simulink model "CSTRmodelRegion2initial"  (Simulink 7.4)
settings: Solver=ode15s  StartTime=0.0  StopTime=500  RelTol=1e-6
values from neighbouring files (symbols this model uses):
  cain = 2    [runDynSim321.m]    (also in sf_CSTR.m = cInVec(1))
  cbin = 1.5    [runDynSim321.m]    (also in sf_CSTR.m = cInVec(2))
undefined symbols (not defined in the file or in its folder): Floor, Ideal, internal, PI, sigbuilder_block
libraries: simulink_extras x2

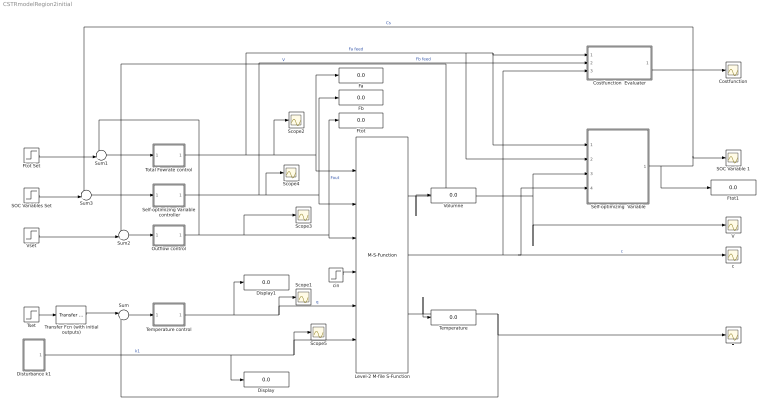
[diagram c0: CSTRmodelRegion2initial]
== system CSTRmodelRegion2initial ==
  Costfunction : Scope
  Costfunction  Evaluater : Subsystem
  Display : Display
  Display1 : Display
  Disturbance k1 : Subsystem
  Fa : Display
  Fb : Display
  Ftot : Display
  Ftot Set : Step  Time=0  Before=22  After=22  SampleTime=0
  Ftot1 : Display
  Level-2 M-file S-Function : M-S-Function  FunctionName=sf_CSTR
  Outflow control : Subsystem  AncestorBlock=simulink/Continuous/PID Controller  DialogController=pidpack.PIDConfig.pidDDGCreate  DialogControllerArgs=DataTag2  mask(PID 1dof){Controller=PI, TimeDomain=Continuous-time, SampleTime=1, IntegratorMethod=Forward Euler, FilterMethod=Forward Euler, Form=Ideal, P=-5, I=0.8, D=0, N=100, InitialConditionSource=internal, InitialConditionForIntegrator=0, InitialConditionForFilter=0, ExternalReset=none, IgnoreLimit=off, ZeroCross=on, LimitOutput=off, UpperSaturationLimit=inf, LowerSaturationLimit=-inf, LinearizeAsGain=off, AntiWindupMode=none, Kb=1, TrackingMode=off, Kt=1, RndMeth=Floor, SaturateOnIntegerOverflow=off, LockScale=off, PParamMin=[], PParamMax=[], PParamDataTypeStr=Inherit: Inherit via internal rule, IParamMin=[], IParamMax=[], IParamDataTypeStr=Inherit: Inherit via internal rule, DParamMin=[], DParamMax=[], DParamDataTypeStr=Inherit: Inherit via internal rule, NParamMin=[], NParamMax=[], NParamDataTypeStr=Inherit: Inherit via internal rule, KbParamMin=[], KbParamMax=[], KbParamDataTypeStr=Inherit: Inherit via internal rule, KtParamMin=[], KtParamMax=[], KtParamDataTypeStr=Inherit: Inherit via internal rule, POutMin=[], POutMax=[], POutDataTypeStr=Inherit: Inherit via internal rule, IOutMin=[], IOutMax=[], IOutDataTypeStr=Inherit: Inherit via internal rule, DOutMin=[], DOutMax=[], DOutDataTypeStr=Inherit: Inherit via internal rule, NOutMin=[], NOutMax=[], NOutDataTypeStr=Inherit: Inherit via internal rule, KbOutMin=[], KbOutMax=[], KbOutDataTypeStr=Inherit: Inherit via internal rule, KtOutMin=[], KtOutMax=[], KtOutDataTypeStr=Inherit: Inherit via internal rule, IntegratorOutMin=[], IntegratorOutMax=[], IntegratorOutDataTypeStr=Inherit: Inherit via internal rule, FilterOutMin=[], FilterOutMax=[], FilterOutDataTypeStr=Inherit: Inherit via internal rule, SumOutMin=[], SumOutMax=[], SumOutDataTypeStr=Inherit: Inherit via internal rule, SumI1OutMin=[], SumI1OutMax=[], SumI1OutDataTypeStr=Inherit: Inherit via internal rule, SumI2OutMin=[], SumI2OutMax=[], SumI2OutDataTypeStr=Inherit: Inherit via internal rule, SumI3OutMin=[], SumI3OutMax=[], SumI3OutDataTypeStr=Inherit: Inherit via internal rule, SumDOutMin=[], SumDOutMax=[], SumDOutDataTypeStr=Inherit: Inherit via internal rule, SumAccumDataTypeStr=Inherit: Inherit via internal rule, SumI1AccumDataTypeStr=Inherit: Inherit via internal rule, SumI2AccumDataTypeStr=Inherit: Inherit via internal rule, SumI3AccumDataTypeStr=Inherit: Inherit via internal rule, SumDAccumDataTypeStr=Inherit: Inherit via internal rule, SaturationOutMin=[], SaturationOutMax=[], SaturationOutDataTypeStr=Inherit: Same as input, IntegratorContinuousStateAttributes='', IntegratorStateIdentifier=, IntegratorStateMustResolveToSignalObject=off, IntegratorRTWStateStorageClass=Auto, IntegratorRTWStateStorageTypeQualifier=, FilterContinuousStateAttributes='', FilterStateIdentifier=, FilterStateMustResolveToSignalObject=off, FilterRTWStateStorageClass=Auto, FilterRTWStateStorageTypeQualifier=}
      mask prompts: TimeDomain "Time-domain:"; SampleTime "Sample time (-1 for inherited):"; IntegratorMethod "Integrator method:"; FilterMethod "Filter method:"; Form "Controller form:"; P "Proportional (P):"; I "Integral (I):"; D "Derivative (D):"; N "Filter coefficient (N):"; InitialConditionSource "Source:"; InitialConditionForIntegrator "Integrator:"; InitialConditionForFilter "Filter:"; ExternalReset "External reset:"; IgnoreLimit "Ignore reset when linearizing"; ZeroCross "Enable zero-crossing detection"; LimitOutput "Limit output"; UpperSaturationLimit "Upper saturation limit:"; LowerSaturationLimit "Lower saturation limit:"; LinearizeAsGain "Ignore saturation when linearizing"; AntiWindupMode "Anti-windup method:"; Kb "Back-calculation coefficient (Kb):"; TrackingMode "Enable tracking mode"; Kt "Tracking coefficient (Kt):"; RndMeth "Integer rounding mode:"; SaturateOnIntegerOverflow "Saturate on integer overflow"; LockScale "Lock data type settings against changes by the fixed-point tools"; PParamMin "P parameter minimum:"; PParamMax "P parameter maximum:"; PParamDataTypeStr "P parameter:"; IParamMin "I parameter minimum:"; IParamMax "I parameter maximum:"; IParamDataTypeStr "I parameter:"; DParamMin "D parameter minimum:"; DParamMax "D parameter maximum:"; DParamDataTypeStr "D parameter:"; NParamMin "N parameter minimum:"; NParamMax "N parameter maximum:"; NParamDataTypeStr "N parameter:"; KbParamMin "Kb parameter minimum:"; KbParamMax "Kb parameter maximum:"; KbParamDataTypeStr "Kb parameter:"; KtParamMin "Kt parameter minimum:"; KtParamMax "Kt parameter maximum:"; KtParamDataTypeStr "Kt parameter:"; POutMin "P product output minimum:"; POutMax "P product output maximum:"; POutDataTypeStr "P product output:"; IOutMin "I product output minimum:"; IOutMax "I product output maximum:"; IOutDataTypeStr "I product output:"; DOutMin "D product output minimum:"; DOutMax "D product output maximum:"; DOutDataTypeStr "D product output:"; NOutMin "N product output minimum:"; NOutMax "N product output maximum:"; NOutDataTypeStr "N product output:"; KbOutMin "Kb product output minimum:"; KbOutMax "Kb product output maximum:"; KbOutDataTypeStr "Kb product output:"; KtOutMin "Kt product output minimum:"; KtOutMax "Kt product output maximum:"; KtOutDataTypeStr "Kt product output:"; IntegratorOutMin "Integrator output minimum:"; IntegratorOutMax "Integrator output maximum:"; IntegratorOutDataTypeStr "Integrator output:"; FilterOutMin "Filter output minimum:"; FilterOutMax "Filter output maximum:"; FilterOutDataTypeStr "Filter output:"; SumOutMin "Sum output minimum:"; SumOutMax "Sum output maximum:"; SumOutDataTypeStr "Sum output:"; SumI1OutMin "SumI1 output minimum:"; SumI1OutMax "SumI1 output maximum:"; SumI1OutDataTypeStr "SumI1 output:"; SumI2OutMin "SumI2 output minimum:"; SumI2OutMax "SumI2 output maximum:"; SumI2OutDataTypeStr "SumI2 output:"; SumI3OutMin "SumI3 output minimum:"; SumI3OutMax "SumI3 output maximum:"; SumI3OutDataTypeStr "SumI3 output:"; SumDOutMin "SumD output minimum:"; SumDOutMax "SumD output maximum:"; SumDOutDataTypeStr "SumD output:"; SumAccumDataTypeStr "Accumulator of Sum:"; SumI1AccumDataTypeStr "Accumulator of SumI1:"; SumI2AccumDataTypeStr "Accumulator of SumI2:"; SumI3AccumDataTypeStr "Accumulator of SumI3:"; SumDAccumDataTypeStr "Accumulator of SumD:"; SaturationOutMin "Saturation output minimum:"; SaturationOutMax "Saturation output maximum:"; SaturationOutDataTypeStr "Saturation output:"; IntegratorContinuousStateAttributes "State name: (e.g., 'position')"; IntegratorStateIdentifier "State name:"; IntegratorStateMustResolveToSignalObject "State name must resolve to Simulink signal object"; IntegratorRTWStateStorageClass "Real-Time Workshop storage class:"; IntegratorRTWStateStorageTypeQualifier "Real-Time Workshop storage type qualifier:"; FilterContinuousStateAttributes "State name: (e.g., 'position')"; FilterStateIdentifier "State name:"; FilterStateMustResolveToSignalObject "State name must resolve to Simulink signal object"; FilterRTWStateStorageClass "Real-Time Workshop storage class:"; FilterRTWStateStorageTypeQualifier "Real-Time Workshop storage type qualifier:"
      mask help: This block implements continuous- and discrete-time PID control algorithms and includes advanced features such as anti-windup, external reset, and signal tracking. You can tune the PID gains automatically using the 'Tune...' button (requires Simulink Control Design).
      mask init:
      | [shiftx shifty satshiftx satshifty] = pidpack.PIDConfig.configPID(gcbh);
  SOC Variable 1 : Scope
  SOC Variables Set : Step  Time=0  After=0  SampleTime=0
  Scope{1..5} (5 alike) : Scope
  Self-optimizing  Variable : Stateflow chart
  Self-optimizing Variable  controller : Subsystem  AncestorBlock=simulink/Continuous/PID Controller  DialogController=pidpack.PIDConfig.pidDDGCreate  DialogControllerArgs=DataTag3  mask(PID 1dof){Controller=PI, TimeDomain=Continuous-time, SampleTime=1, IntegratorMethod=Forward Euler, FilterMethod=Forward Euler, Form=Ideal, P=145, I=3, D=0, N=100, InitialConditionSource=internal, InitialConditionForIntegrator=0, InitialConditionForFilter=0, ExternalReset=none, IgnoreLimit=off, ZeroCross=on, LimitOutput=off, UpperSaturationLimit=1e6, LowerSaturationLimit=0, LinearizeAsGain=off, AntiWindupMode=none, Kb=1, TrackingMode=off, Kt=1, RndMeth=Floor, SaturateOnIntegerOverflow=off, LockScale=off, PParamMin=[], PParamMax=[], PParamDataTypeStr=Inherit: Inherit via internal rule, IParamMin=[], IParamMax=[], IParamDataTypeStr=Inherit: Inherit via internal rule, DParamMin=[], DParamMax=[], DParamDataTypeStr=Inherit: Inherit via internal rule, NParamMin=[], NParamMax=[], NParamDataTypeStr=Inherit: Inherit via internal rule, KbParamMin=[], KbParamMax=[], KbParamDataTypeStr=Inherit: Inherit via internal rule, KtParamMin=[], KtParamMax=[], KtParamDataTypeStr=Inherit: Inherit via internal rule, POutMin=[], POutMax=[], POutDataTypeStr=Inherit: Inherit via internal rule, IOutMin=[], IOutMax=[], IOutDataTypeStr=Inherit: Inherit via internal rule, DOutMin=[], DOutMax=[], DOutDataTypeStr=Inherit: Inherit via internal rule, NOutMin=[], NOutMax=[], NOutDataTypeStr=Inherit: Inherit via internal rule, KbOutMin=[], KbOutMax=[], KbOutDataTypeStr=Inherit: Inherit via internal rule, KtOutMin=[], KtOutMax=[], KtOutDataTypeStr=Inherit: Inherit via internal rule, IntegratorOutMin=[], IntegratorOutMax=[], IntegratorOutDataTypeStr=Inherit: Inherit via internal rule, FilterOutMin=[], FilterOutMax=[], FilterOutDataTypeStr=Inherit: Inherit via internal rule, SumOutMin=[], SumOutMax=[], SumOutDataTypeStr=Inherit: Inherit via internal rule, SumI1OutMin=[], SumI1OutMax=[], SumI1OutDataTypeStr=Inherit: Inherit via internal rule, SumI2OutMin=[], SumI2OutMax=[], SumI2OutDataTypeStr=Inherit: Inherit via internal rule, SumI3OutMin=[], SumI3OutMax=[], SumI3OutDataTypeStr=Inherit: Inherit via internal rule, SumDOutMin=[], SumDOutMax=[], SumDOutDataTypeStr=Inherit: Inherit via internal rule, SumAccumDataTypeStr=Inherit: Inherit via internal rule, SumI1AccumDataTypeStr=Inherit: Inherit via internal rule, SumI2AccumDataTypeStr=Inherit: Inherit via internal rule, SumI3AccumDataTypeStr=Inherit: Inherit via internal rule, SumDAccumDataTypeStr=Inherit: Inherit via internal rule, SaturationOutMin=[], SaturationOutMax=[], SaturationOutDataTypeStr=Inherit: Same as input, IntegratorContinuousStateAttributes='', IntegratorStateIdentifier=, IntegratorStateMustResolveToSignalObject=off, IntegratorRTWStateStorageClass=Auto, IntegratorRTWStateStorageTypeQualifier=, FilterContinuousStateAttributes='', FilterStateIdentifier=, FilterStateMustResolveToSignalObject=off, FilterRTWStateStorageClass=Auto, FilterRTWStateStorageTypeQualifier=}
      mask prompts: TimeDomain "Time-domain:"; SampleTime "Sample time (-1 for inherited):"; IntegratorMethod "Integrator method:"; FilterMethod "Filter method:"; Form "Controller form:"; P "Proportional (P):"; I "Integral (I):"; D "Derivative (D):"; N "Filter coefficient (N):"; InitialConditionSource "Source:"; InitialConditionForIntegrator "Integrator:"; InitialConditionForFilter "Filter:"; ExternalReset "External reset:"; IgnoreLimit "Ignore reset when linearizing"; ZeroCross "Enable zero-crossing detection"; LimitOutput "Limit output"; UpperSaturationLimit "Upper saturation limit:"; LowerSaturationLimit "Lower saturation limit:"; LinearizeAsGain "Ignore saturation when linearizing"; AntiWindupMode "Anti-windup method:"; Kb "Back-calculation coefficient (Kb):"; TrackingMode "Enable tracking mode"; Kt "Tracking coefficient (Kt):"; RndMeth "Integer rounding mode:"; SaturateOnIntegerOverflow "Saturate on integer overflow"; LockScale "Lock data type settings against changes by the fixed-point tools"; PParamMin "P parameter minimum:"; PParamMax "P parameter maximum:"; PParamDataTypeStr "P parameter:"; IParamMin "I parameter minimum:"; IParamMax "I parameter maximum:"; IParamDataTypeStr "I parameter:"; DParamMin "D parameter minimum:"; DParamMax "D parameter maximum:"; DParamDataTypeStr "D parameter:"; NParamMin "N parameter minimum:"; NParamMax "N parameter maximum:"; NParamDataTypeStr "N parameter:"; KbParamMin "Kb parameter minimum:"; KbParamMax "Kb parameter maximum:"; KbParamDataTypeStr "Kb parameter:"; KtParamMin "Kt parameter minimum:"; KtParamMax "Kt parameter maximum:"; KtParamDataTypeStr "Kt parameter:"; POutMin "P product output minimum:"; POutMax "P product output maximum:"; POutDataTypeStr "P product output:"; IOutMin "I product output minimum:"; IOutMax "I product output maximum:"; IOutDataTypeStr "I product output:"; DOutMin "D product output minimum:"; DOutMax "D product output maximum:"; DOutDataTypeStr "D product output:"; NOutMin "N product output minimum:"; NOutMax "N product output maximum:"; NOutDataTypeStr "N product output:"; KbOutMin "Kb product output minimum:"; KbOutMax "Kb product output maximum:"; KbOutDataTypeStr "Kb product output:"; KtOutMin "Kt product output minimum:"; KtOutMax "Kt product output maximum:"; KtOutDataTypeStr "Kt product output:"; IntegratorOutMin "Integrator output minimum:"; IntegratorOutMax "Integrator output maximum:"; IntegratorOutDataTypeStr "Integrator output:"; FilterOutMin "Filter output minimum:"; FilterOutMax "Filter output maximum:"; FilterOutDataTypeStr "Filter output:"; SumOutMin "Sum output minimum:"; SumOutMax "Sum output maximum:"; SumOutDataTypeStr "Sum output:"; SumI1OutMin "SumI1 output minimum:"; SumI1OutMax "SumI1 output maximum:"; SumI1OutDataTypeStr "SumI1 output:"; SumI2OutMin "SumI2 output minimum:"; SumI2OutMax "SumI2 output maximum:"; SumI2OutDataTypeStr "SumI2 output:"; SumI3OutMin "SumI3 output minimum:"; SumI3OutMax "SumI3 output maximum:"; SumI3OutDataTypeStr "SumI3 output:"; SumDOutMin "SumD output minimum:"; SumDOutMax "SumD output maximum:"; SumDOutDataTypeStr "SumD output:"; SumAccumDataTypeStr "Accumulator of Sum:"; SumI1AccumDataTypeStr "Accumulator of SumI1:"; SumI2AccumDataTypeStr "Accumulator of SumI2:"; SumI3AccumDataTypeStr "Accumulator of SumI3:"; SumDAccumDataTypeStr "Accumulator of SumD:"; SaturationOutMin "Saturation output minimum:"; SaturationOutMax "Saturation output maximum:"; SaturationOutDataTypeStr "Saturation output:"; IntegratorContinuousStateAttributes "State name: (e.g., 'position')"; IntegratorStateIdentifier "State name:"; IntegratorStateMustResolveToSignalObject "State name must resolve to Simulink signal object"; IntegratorRTWStateStorageClass "Real-Time Workshop storage class:"; IntegratorRTWStateStorageTypeQualifier "Real-Time Workshop storage type qualifier:"; FilterContinuousStateAttributes "State name: (e.g., 'position')"; FilterStateIdentifier "State name:"; FilterStateMustResolveToSignalObject "State name must resolve to Simulink signal object"; FilterRTWStateStorageClass "Real-Time Workshop storage class:"; FilterRTWStateStorageTypeQualifier "Real-Time Workshop storage type qualifier:"
      mask help: This block implements continuous- and discrete-time PID control algorithms and includes advanced features such as anti-windup, external reset, and signal tracking. You can tune the PID gains automatically using the 'Tune...' button (requires Simulink Control Design).
      mask init:
      | [shiftx shifty satshiftx satshifty] = pidpack.PIDConfig.configPID(gcbh);
  Sum : Sum  Inputs=|+-  OutDataType=fixdt(1, 16)  OutScaling=2^0
  Sum1 : Sum  Inputs=-+|  OutDataType=fixdt(1, 16)  OutScaling=2^0
  Sum2 : Sum  Inputs=-+|  OutDataType=fixdt(1, 16)  OutScaling=2^0
  Sum3 : Sum  Inputs=-+|  OutDataType=fixdt(1, 16)  OutScaling=2^0
  T : Scope
  Temperature : Display
  Temperature control : Subsystem  AncestorBlock=simulink/Continuous/PID Controller  DialogController=pidpack.PIDConfig.pidDDGCreate  DialogControllerArgs=DataTag4  mask(PID 1dof){Controller=PI, TimeDomain=Continuous-time, SampleTime=1, IntegratorMethod=Forward Euler, FilterMethod=Forward Euler, Form=Ideal, P=-3521, I=2.4, D=0, N=100, InitialConditionSource=internal, InitialConditionForIntegrator=888, InitialConditionForFilter=0, ExternalReset=none, IgnoreLimit=off, ZeroCross=on, LimitOutput=off, UpperSaturationLimit=1e3, LowerSaturationLimit=0, LinearizeAsGain=off, AntiWindupMode=none, Kb=1, TrackingMode=off, Kt=1, RndMeth=Floor, SaturateOnIntegerOverflow=off, LockScale=off, PParamMin=[], PParamMax=[], PParamDataTypeStr=Inherit: Inherit via internal rule, IParamMin=[], IParamMax=[], IParamDataTypeStr=Inherit: Inherit via internal rule, DParamMin=[], DParamMax=[], DParamDataTypeStr=Inherit: Inherit via internal rule, NParamMin=[], NParamMax=[], NParamDataTypeStr=Inherit: Inherit via internal rule, KbParamMin=[], KbParamMax=[], KbParamDataTypeStr=Inherit: Inherit via internal rule, KtParamMin=[], KtParamMax=[], KtParamDataTypeStr=Inherit: Inherit via internal rule, POutMin=[], POutMax=[], POutDataTypeStr=Inherit: Inherit via internal rule, IOutMin=[], IOutMax=[], IOutDataTypeStr=Inherit: Inherit via internal rule, DOutMin=[], DOutMax=[], DOutDataTypeStr=Inherit: Inherit via internal rule, NOutMin=[], NOutMax=[], NOutDataTypeStr=Inherit: Inherit via internal rule, KbOutMin=[], KbOutMax=[], KbOutDataTypeStr=Inherit: Inherit via internal rule, KtOutMin=[], KtOutMax=[], KtOutDataTypeStr=Inherit: Inherit via internal rule, IntegratorOutMin=[], IntegratorOutMax=[], IntegratorOutDataTypeStr=Inherit: Inherit via internal rule, FilterOutMin=[], FilterOutMax=[], FilterOutDataTypeStr=Inherit: Inherit via internal rule, SumOutMin=[], SumOutMax=[], SumOutDataTypeStr=Inherit: Inherit via internal rule, SumI1OutMin=[], SumI1OutMax=[], SumI1OutDataTypeStr=Inherit: Inherit via internal rule, SumI2OutMin=[], SumI2OutMax=[], SumI2OutDataTypeStr=Inherit: Inherit via internal rule, SumI3OutMin=[], SumI3OutMax=[], SumI3OutDataTypeStr=Inherit: Inherit via internal rule, SumDOutMin=[], SumDOutMax=[], SumDOutDataTypeStr=Inherit: Inherit via internal rule, SumAccumDataTypeStr=Inherit: Inherit via internal rule, SumI1AccumDataTypeStr=Inherit: Inherit via internal rule, SumI2AccumDataTypeStr=Inherit: Inherit via internal rule, SumI3AccumDataTypeStr=Inherit: Inherit via internal rule, SumDAccumDataTypeStr=Inherit: Inherit via internal rule, SaturationOutMin=[], SaturationOutMax=[], SaturationOutDataTypeStr=Inherit: Same as input, IntegratorContinuousStateAttributes='', IntegratorStateIdentifier=, IntegratorStateMustResolveToSignalObject=off, IntegratorRTWStateStorageClass=Auto, IntegratorRTWStateStorageTypeQualifier=, FilterContinuousStateAttributes='', FilterStateIdentifier=, FilterStateMustResolveToSignalObject=off, FilterRTWStateStorageClass=Auto, FilterRTWStateStorageTypeQualifier=}
      mask prompts: TimeDomain "Time-domain:"; SampleTime "Sample time (-1 for inherited):"; IntegratorMethod "Integrator method:"; FilterMethod "Filter method:"; Form "Controller form:"; P "Proportional (P):"; I "Integral (I):"; D "Derivative (D):"; N "Filter coefficient (N):"; InitialConditionSource "Source:"; InitialConditionForIntegrator "Integrator:"; InitialConditionForFilter "Filter:"; ExternalReset "External reset:"; IgnoreLimit "Ignore reset when linearizing"; ZeroCross "Enable zero-crossing detection"; LimitOutput "Limit output"; UpperSaturationLimit "Upper saturation limit:"; LowerSaturationLimit "Lower saturation limit:"; LinearizeAsGain "Ignore saturation when linearizing"; AntiWindupMode "Anti-windup method:"; Kb "Back-calculation coefficient (Kb):"; TrackingMode "Enable tracking mode"; Kt "Tracking coefficient (Kt):"; RndMeth "Integer rounding mode:"; SaturateOnIntegerOverflow "Saturate on integer overflow"; LockScale "Lock data type settings against changes by the fixed-point tools"; PParamMin "P parameter minimum:"; PParamMax "P parameter maximum:"; PParamDataTypeStr "P parameter:"; IParamMin "I parameter minimum:"; IParamMax "I parameter maximum:"; IParamDataTypeStr "I parameter:"; DParamMin "D parameter minimum:"; DParamMax "D parameter maximum:"; DParamDataTypeStr "D parameter:"; NParamMin "N parameter minimum:"; NParamMax "N parameter maximum:"; NParamDataTypeStr "N parameter:"; KbParamMin "Kb parameter minimum:"; KbParamMax "Kb parameter maximum:"; KbParamDataTypeStr "Kb parameter:"; KtParamMin "Kt parameter minimum:"; KtParamMax "Kt parameter maximum:"; KtParamDataTypeStr "Kt parameter:"; POutMin "P product output minimum:"; POutMax "P product output maximum:"; POutDataTypeStr "P product output:"; IOutMin "I product output minimum:"; IOutMax "I product output maximum:"; IOutDataTypeStr "I product output:"; DOutMin "D product output minimum:"; DOutMax "D product output maximum:"; DOutDataTypeStr "D product output:"; NOutMin "N product output minimum:"; NOutMax "N product output maximum:"; NOutDataTypeStr "N product output:"; KbOutMin "Kb product output minimum:"; KbOutMax "Kb product output maximum:"; KbOutDataTypeStr "Kb product output:"; KtOutMin "Kt product output minimum:"; KtOutMax "Kt product output maximum:"; KtOutDataTypeStr "Kt product output:"; IntegratorOutMin "Integrator output minimum:"; IntegratorOutMax "Integrator output maximum:"; IntegratorOutDataTypeStr "Integrator output:"; FilterOutMin "Filter output minimum:"; FilterOutMax "Filter output maximum:"; FilterOutDataTypeStr "Filter output:"; SumOutMin "Sum output minimum:"; SumOutMax "Sum output maximum:"; SumOutDataTypeStr "Sum output:"; SumI1OutMin "SumI1 output minimum:"; SumI1OutMax "SumI1 output maximum:"; SumI1OutDataTypeStr "SumI1 output:"; SumI2OutMin "SumI2 output minimum:"; SumI2OutMax "SumI2 output maximum:"; SumI2OutDataTypeStr "SumI2 output:"; SumI3OutMin "SumI3 output minimum:"; SumI3OutMax "SumI3 output maximum:"; SumI3OutDataTypeStr "SumI3 output:"; SumDOutMin "SumD output minimum:"; SumDOutMax "SumD output maximum:"; SumDOutDataTypeStr "SumD output:"; SumAccumDataTypeStr "Accumulator of Sum:"; SumI1AccumDataTypeStr "Accumulator of SumI1:"; SumI2AccumDataTypeStr "Accumulator of SumI2:"; SumI3AccumDataTypeStr "Accumulator of SumI3:"; SumDAccumDataTypeStr "Accumulator of SumD:"; SaturationOutMin "Saturation output minimum:"; SaturationOutMax "Saturation output maximum:"; SaturationOutDataTypeStr "Saturation output:"; IntegratorContinuousStateAttributes "State name: (e.g., 'position')"; IntegratorStateIdentifier "State name:"; IntegratorStateMustResolveToSignalObject "State name must resolve to Simulink signal object"; IntegratorRTWStateStorageClass "Real-Time Workshop storage class:"; IntegratorRTWStateStorageTypeQualifier "Real-Time Workshop storage type qualifier:"; FilterContinuousStateAttributes "State name: (e.g., 'position')"; FilterStateIdentifier "State name:"; FilterStateMustResolveToSignalObject "State name must resolve to Simulink signal object"; FilterRTWStateStorageClass "Real-Time Workshop storage class:"; FilterRTWStateStorageTypeQualifier "Real-Time Workshop storage type qualifier:"
      mask help: This block implements continuous- and discrete-time PID control algorithms and includes advanced features such as anti-windup, external reset, and signal tracking. You can tune the PID gains automatically using the 'Tune...' button (requires Simulink Control Design).
      mask init:
      | [shiftx shifty satshiftx satshifty] = pidpack.PIDConfig.configPID(gcbh);
  Total Fowrate control : Subsystem  AncestorBlock=simulink/Continuous/PID Controller  DialogController=pidpack.PIDConfig.pidDDGCreate  DialogControllerArgs=DataTag5  mask(PID 1dof){Controller=PI, TimeDomain=Continuous-time, SampleTime=1, IntegratorMethod=Forward Euler, FilterMethod=Forward Euler, Form=Ideal, P=0.58, I=0.35, D=0, N=100, InitialConditionSource=internal, InitialConditionForIntegrator=0, InitialConditionForFilter=0, ExternalReset=none, IgnoreLimit=off, ZeroCross=on, LimitOutput=off, UpperSaturationLimit=1e6, LowerSaturationLimit=0, LinearizeAsGain=off, AntiWindupMode=none, Kb=1, TrackingMode=off, Kt=1, RndMeth=Floor, SaturateOnIntegerOverflow=off, LockScale=off, PParamMin=[], PParamMax=[], PParamDataTypeStr=Inherit: Inherit via internal rule, IParamMin=[], IParamMax=[], IParamDataTypeStr=Inherit: Inherit via internal rule, DParamMin=[], DParamMax=[], DParamDataTypeStr=Inherit: Inherit via internal rule, NParamMin=[], NParamMax=[], NParamDataTypeStr=Inherit: Inherit via internal rule, KbParamMin=[], KbParamMax=[], KbParamDataTypeStr=Inherit: Inherit via internal rule, KtParamMin=[], KtParamMax=[], KtParamDataTypeStr=Inherit: Inherit via internal rule, POutMin=[], POutMax=[], POutDataTypeStr=Inherit: Inherit via internal rule, IOutMin=[], IOutMax=[], IOutDataTypeStr=Inherit: Inherit via internal rule, DOutMin=[], DOutMax=[], DOutDataTypeStr=Inherit: Inherit via internal rule, NOutMin=[], NOutMax=[], NOutDataTypeStr=Inherit: Inherit via internal rule, KbOutMin=[], KbOutMax=[], KbOutDataTypeStr=Inherit: Inherit via internal rule, KtOutMin=[], KtOutMax=[], KtOutDataTypeStr=Inherit: Inherit via internal rule, IntegratorOutMin=[], IntegratorOutMax=[], IntegratorOutDataTypeStr=Inherit: Inherit via internal rule, FilterOutMin=[], FilterOutMax=[], FilterOutDataTypeStr=Inherit: Inherit via internal rule, SumOutMin=[], SumOutMax=[], SumOutDataTypeStr=Inherit: Inherit via internal rule, SumI1OutMin=[], SumI1OutMax=[], SumI1OutDataTypeStr=Inherit: Inherit via internal rule, SumI2OutMin=[], SumI2OutMax=[], SumI2OutDataTypeStr=Inherit: Inherit via internal rule, SumI3OutMin=[], SumI3OutMax=[], SumI3OutDataTypeStr=Inherit: Inherit via internal rule, SumDOutMin=[], SumDOutMax=[], SumDOutDataTypeStr=Inherit: Inherit via internal rule, SumAccumDataTypeStr=Inherit: Inherit via internal rule, SumI1AccumDataTypeStr=Inherit: Inherit via internal rule, SumI2AccumDataTypeStr=Inherit: Inherit via internal rule, SumI3AccumDataTypeStr=Inherit: Inherit via internal rule, SumDAccumDataTypeStr=Inherit: Inherit via internal rule, SaturationOutMin=[], SaturationOutMax=[], SaturationOutDataTypeStr=Inherit: Same as input, IntegratorContinuousStateAttributes='', IntegratorStateIdentifier=, IntegratorStateMustResolveToSignalObject=off, IntegratorRTWStateStorageClass=Auto, IntegratorRTWStateStorageTypeQualifier=, FilterContinuousStateAttributes='', FilterStateIdentifier=, FilterStateMustResolveToSignalObject=off, FilterRTWStateStorageClass=Auto, FilterRTWStateStorageTypeQualifier=}
      mask prompts: TimeDomain "Time-domain:"; SampleTime "Sample time (-1 for inherited):"; IntegratorMethod "Integrator method:"; FilterMethod "Filter method:"; Form "Controller form:"; P "Proportional (P):"; I "Integral (I):"; D "Derivative (D):"; N "Filter coefficient (N):"; InitialConditionSource "Source:"; InitialConditionForIntegrator "Integrator:"; InitialConditionForFilter "Filter:"; ExternalReset "External reset:"; IgnoreLimit "Ignore reset when linearizing"; ZeroCross "Enable zero-crossing detection"; LimitOutput "Limit output"; UpperSaturationLimit "Upper saturation limit:"; LowerSaturationLimit "Lower saturation limit:"; LinearizeAsGain "Ignore saturation when linearizing"; AntiWindupMode "Anti-windup method:"; Kb "Back-calculation coefficient (Kb):"; TrackingMode "Enable tracking mode"; Kt "Tracking coefficient (Kt):"; RndMeth "Integer rounding mode:"; SaturateOnIntegerOverflow "Saturate on integer overflow"; LockScale "Lock data type settings against changes by the fixed-point tools"; PParamMin "P parameter minimum:"; PParamMax "P parameter maximum:"; PParamDataTypeStr "P parameter:"; IParamMin "I parameter minimum:"; IParamMax "I parameter maximum:"; IParamDataTypeStr "I parameter:"; DParamMin "D parameter minimum:"; DParamMax "D parameter maximum:"; DParamDataTypeStr "D parameter:"; NParamMin "N parameter minimum:"; NParamMax "N parameter maximum:"; NParamDataTypeStr "N parameter:"; KbParamMin "Kb parameter minimum:"; KbParamMax "Kb parameter maximum:"; KbParamDataTypeStr "Kb parameter:"; KtParamMin "Kt parameter minimum:"; KtParamMax "Kt parameter maximum:"; KtParamDataTypeStr "Kt parameter:"; POutMin "P product output minimum:"; POutMax "P product output maximum:"; POutDataTypeStr "P product output:"; IOutMin "I product output minimum:"; IOutMax "I product output maximum:"; IOutDataTypeStr "I product output:"; DOutMin "D product output minimum:"; DOutMax "D product output maximum:"; DOutDataTypeStr "D product output:"; NOutMin "N product output minimum:"; NOutMax "N product output maximum:"; NOutDataTypeStr "N product output:"; KbOutMin "Kb product output minimum:"; KbOutMax "Kb product output maximum:"; KbOutDataTypeStr "Kb product output:"; KtOutMin "Kt product output minimum:"; KtOutMax "Kt product output maximum:"; KtOutDataTypeStr "Kt product output:"; IntegratorOutMin "Integrator output minimum:"; IntegratorOutMax "Integrator output maximum:"; IntegratorOutDataTypeStr "Integrator output:"; FilterOutMin "Filter output minimum:"; FilterOutMax "Filter output maximum:"; FilterOutDataTypeStr "Filter output:"; SumOutMin "Sum output minimum:"; SumOutMax "Sum output maximum:"; SumOutDataTypeStr "Sum output:"; SumI1OutMin "SumI1 output minimum:"; SumI1OutMax "SumI1 output maximum:"; SumI1OutDataTypeStr "SumI1 output:"; SumI2OutMin "SumI2 output minimum:"; SumI2OutMax "SumI2 output maximum:"; SumI2OutDataTypeStr "SumI2 output:"; SumI3OutMin "SumI3 output minimum:"; SumI3OutMax "SumI3 output maximum:"; SumI3OutDataTypeStr "SumI3 output:"; SumDOutMin "SumD output minimum:"; SumDOutMax "SumD output maximum:"; SumDOutDataTypeStr "SumD output:"; SumAccumDataTypeStr "Accumulator of Sum:"; SumI1AccumDataTypeStr "Accumulator of SumI1:"; SumI2AccumDataTypeStr "Accumulator of SumI2:"; SumI3AccumDataTypeStr "Accumulator of SumI3:"; SumDAccumDataTypeStr "Accumulator of SumD:"; SaturationOutMin "Saturation output minimum:"; SaturationOutMax "Saturation output maximum:"; SaturationOutDataTypeStr "Saturation output:"; IntegratorContinuousStateAttributes "State name: (e.g., 'position')"; IntegratorStateIdentifier "State name:"; IntegratorStateMustResolveToSignalObject "State name must resolve to Simulink signal object"; IntegratorRTWStateStorageClass "Real-Time Workshop storage class:"; IntegratorRTWStateStorageTypeQualifier "Real-Time Workshop storage type qualifier:"; FilterContinuousStateAttributes "State name: (e.g., 'position')"; FilterStateIdentifier "State name:"; FilterStateMustResolveToSignalObject "State name must resolve to Simulink signal object"; FilterRTWStateStorageClass "Real-Time Workshop storage class:"; FilterRTWStateStorageTypeQualifier "Real-Time Workshop storage type qualifier:"
      mask help: This block implements continuous- and discrete-time PID control algorithms and includes advanced features such as anti-windup, external reset, and signal tracking. You can tune the PID gains automatically using the 'Tune...' button (requires Simulink Control Design).
      mask init:
      | [shiftx shifty satshiftx satshifty] = pidpack.PIDConfig.configPID(gcbh);
  Transfer Fcn (with initial outputs) : simulink_extras/Additional Linear/Transfer Fcn (with initial outputs)  SystemSampleTime=-1  N=[1]  D="[10  1]"  Y0=350  U0=0
  Tset : Step  Time=250  Before=350  After=350  SampleTime=0
  V : Scope
  Volumne : Display
  Vset : Step  Time=0  Before=500  After=500  SampleTime=0
  c : Scope
  cin : Step  Time=0  Before=[cain cbin 0 0]  After=[cain cbin 0 0]  SampleTime=0
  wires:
  cin/1 -> Level-2 M-file S-Function/4
  Sum/1 -> Temperature control/1(u)
  Level-2 M-file S-Function/1 -> Sum2/1, Self-optimizing  Variable/3(V), V/1, Volumne/1  "V"
  Level-2 M-file S-Function/2 -> Costfunction  Evaluater/3(Concentrations), c/1, Self-optimizing  Variable/4(cVector)  "c"
  Level-2 M-file S-Function/3 -> T/1, Sum/2, Temperature/1  "T"
  Tset/1 -> Transfer Fcn (with initial outputs)/1
  Vset/1 -> Sum2/2
  Sum2/1 -> Outflow control/1(u)
  Costfunction  Evaluater/1(Objective) -> Costfunction/1
  Outflow control/1(y) -> Scope3/1, Level-2 M-file S-Function/3, Ftot/1, Sum1/1  "Fout"
  Temperature control/1(y) -> Level-2 M-file S-Function/5, Scope1/1, Display1/1  "q"
  Sum1/1 -> Total Fowrate control/1(u)
  Total Fowrate control/1(y) -> Scope2/1, Level-2 M-file S-Function/1, Fa/1, Costfunction  Evaluater/1(Fa), Self-optimizing  Variable/1(Fa), Self-optimizing  Variable/2(Fb)  "Fa feed"
  Self-optimizing  Variable/1(cs) -> SOC Variable 1/1, Sum3/1, Ftot1/1  "Cs"
  SOC Variables Set/1 -> Sum3/2
  Sum3/1 -> Self-optimizing Variable  controller/1(u)
  Self-optimizing Variable  controller/1(y) -> Costfunction  Evaluater/2(Fb), Scope4/1, Level-2 M-file S-Function/2, Fb/1  "Fb feed"
  Ftot Set/1 -> Sum1/2
  Disturbance k1/1(Out1) -> Level-2 M-file S-Function/6, Scope5/1, Display/1  "k1"
  Transfer Fcn (with initial outputs)/1 -> Sum/1

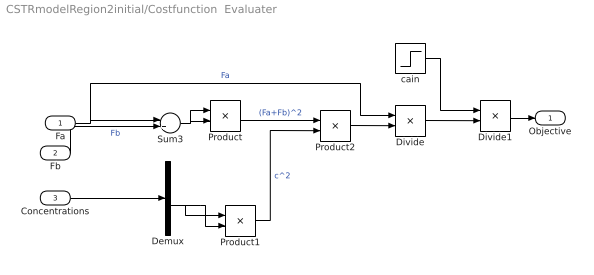
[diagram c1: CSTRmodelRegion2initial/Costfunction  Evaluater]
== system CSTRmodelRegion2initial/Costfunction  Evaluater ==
  Fa : Inport
  Fb : Inport  Port=2
  Concentrations : Inport  Port=3
  Demux : Demux
  Divide : Product  Inputs=/*  OutDataType=fixdt(1, 16)  OutScaling=2^-10
  Divide1 : Product  Inputs=/*  OutDataType=fixdt(1, 16)  OutScaling=2^-10
  Product : Product  OutDataType=fixdt(1, 16)  OutScaling=2^0
  Product1 : Product  OutDataType=fixdt(1, 16)  OutScaling=2^0
  Product2 : Product  OutDataType=fixdt(1, 16)  OutScaling=2^0
  Sum3 : Sum  Inputs=|++  OutDataType=fixdt(1, 16)  OutScaling=2^0
  cain : Step  Before=cain  After=cain  SampleTime=0
  Objective : Outport
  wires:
  Sum3/1 -> Product/1, Product/2
  Demux/3 -> Product1/2, Product1/1
  Product/1 -> Product2/1  "(Fa+Fb)^2"
  Product1/1 -> Product2/2  "c^2"
  Product2/1 -> Divide/2
  Divide/1 -> Divide1/2
  cain/1 -> Divide1/1
  Fa/1 -> Sum3/1, Divide/1  "Fa"
  Fb/1 -> Sum3/2  "Fb"
  Concentrations/1 -> Demux/1
  Divide1/1 -> Objective/1
  Demux/1 -> ?
  Demux/2 -> ?
  Demux/4 -> ?

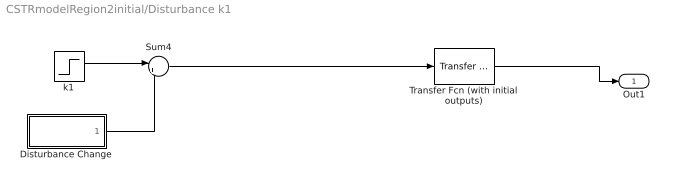
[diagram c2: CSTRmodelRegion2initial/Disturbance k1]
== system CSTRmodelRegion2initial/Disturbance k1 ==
  Disturbance Change : Subsystem  Tag=STV Subsys  LoadFcn=sigbuilder_block('load',[0.8 12.8 1534.4 831.2 ]);  StartFcn=sigbuilder_block('start');  StopFcn=sigbuilder_block('stop');  ClipboardFcn=sigbuilder_block('clipboard');
  Sum4 : Sum  Inputs=|++  OutDataType=fixdt(1, 16)  OutScaling=2^0
  Transfer Fcn (with initial outputs) : simulink_extras/Additional Linear/Transfer Fcn (with initial outputs)  SystemSampleTime=-1  N=[1]  D="[20  1]"  Y0=0  U0=0
  k1 : Step  Time=200  Before=0.3  After=0.3  SampleTime=0
  Out1 : Outport
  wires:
  k1/1 -> Sum4/1
  Sum4/1 -> Transfer Fcn (with initial outputs)/1
  Transfer Fcn (with initial outputs)/1 -> Out1/1
  Disturbance Change/1(Signal 1) -> Sum4/2

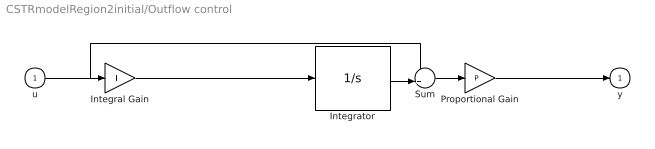
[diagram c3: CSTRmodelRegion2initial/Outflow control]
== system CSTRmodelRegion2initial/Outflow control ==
  u : Inport  OutDataType=OutDataTypeStr
  Integral Gain : Gain  DisableCoverage=on  Gain=I  ParamMin=IParamMin  ParamMax=IParamMax  ParameterDataTypeMode=Specify via dialog  ParameterDataType=IParamDataTypeStr  ParamDataTypeStr=IParamDataTypeStr  OutMin=IOutMin  OutMax=IOutMax  OutDataTypeMode=Specify via dialog  OutDataType=IOutDataTypeStr  OutDataTypeStr=IOutDataTypeStr
  Integrator : Integrator  DisableCoverage=on  InitialCondition=InitialConditionForIntegrator
  Proportional Gain : Gain  Gain=P  ParamMin=PParamMin  ParamMax=PParamMax  ParameterDataTypeMode=Specify via dialog  ParameterDataType=PParamDataTypeStr  ParamDataTypeStr=PParamDataTypeStr  OutMin=POutMin  OutMax=POutMax  OutDataTypeMode=Specify via dialog  OutDataType=POutDataTypeStr  OutDataTypeStr=POutDataTypeStr
  Sum : Sum  DisableCoverage=on  Inputs=++|  AccumDataTypeStr=SumAccumDataTypeStr  OutMin=SumOutMin  OutMax=SumOutMax  OutDataTypeMode=Specify via dialog  OutDataType=SumOutDataTypeStr  OutDataTypeStr=SumOutDataTypeStr
  y : Outport  OutDataType=OutDataTypeStr  InitialOutput=0
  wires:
  u/1 -> Sum/1, Integral Gain/1
  Proportional Gain/1 -> y/1
  Integral Gain/1 -> Integrator/1
  Integrator/1 -> Sum/2
  Sum/1 -> Proportional Gain/1

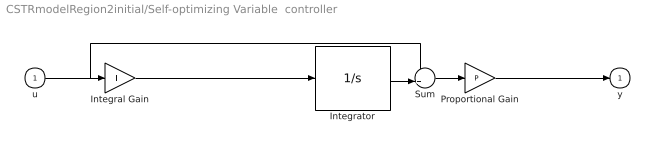
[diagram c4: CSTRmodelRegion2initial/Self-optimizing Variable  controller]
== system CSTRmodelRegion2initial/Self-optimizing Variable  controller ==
  u : Inport  OutDataType=OutDataTypeStr
  Integral Gain : Gain  DisableCoverage=on  Gain=I  ParamMin=IParamMin  ParamMax=IParamMax  ParameterDataTypeMode=Specify via dialog  ParameterDataType=IParamDataTypeStr  ParamDataTypeStr=IParamDataTypeStr  OutMin=IOutMin  OutMax=IOutMax  OutDataTypeMode=Specify via dialog  OutDataType=IOutDataTypeStr  OutDataTypeStr=IOutDataTypeStr
  Integrator : Integrator  DisableCoverage=on  InitialCondition=InitialConditionForIntegrator
  Proportional Gain : Gain  Gain=P  ParamMin=PParamMin  ParamMax=PParamMax  ParameterDataTypeMode=Specify via dialog  ParameterDataType=PParamDataTypeStr  ParamDataTypeStr=PParamDataTypeStr  OutMin=POutMin  OutMax=POutMax  OutDataTypeMode=Specify via dialog  OutDataType=POutDataTypeStr  OutDataTypeStr=POutDataTypeStr
  Sum : Sum  DisableCoverage=on  Inputs=++|  AccumDataTypeStr=SumAccumDataTypeStr  OutMin=SumOutMin  OutMax=SumOutMax  OutDataTypeMode=Specify via dialog  OutDataType=SumOutDataTypeStr  OutDataTypeStr=SumOutDataTypeStr
  y : Outport  OutDataType=OutDataTypeStr  InitialOutput=0
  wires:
  u/1 -> Sum/1, Integral Gain/1
  Proportional Gain/1 -> y/1
  Integral Gain/1 -> Integrator/1
  Integrator/1 -> Sum/2
  Sum/1 -> Proportional Gain/1

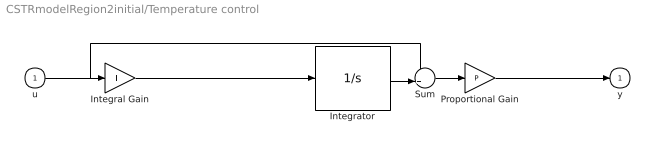
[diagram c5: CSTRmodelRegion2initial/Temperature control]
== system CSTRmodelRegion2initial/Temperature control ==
  u : Inport  OutDataType=OutDataTypeStr
  Integral Gain : Gain  DisableCoverage=on  Gain=I  ParamMin=IParamMin  ParamMax=IParamMax  ParameterDataTypeMode=Specify via dialog  ParameterDataType=IParamDataTypeStr  ParamDataTypeStr=IParamDataTypeStr  OutMin=IOutMin  OutMax=IOutMax  OutDataTypeMode=Specify via dialog  OutDataType=IOutDataTypeStr  OutDataTypeStr=IOutDataTypeStr
  Integrator : Integrator  DisableCoverage=on  InitialCondition=InitialConditionForIntegrator
  Proportional Gain : Gain  Gain=P  ParamMin=PParamMin  ParamMax=PParamMax  ParameterDataTypeMode=Specify via dialog  ParameterDataType=PParamDataTypeStr  ParamDataTypeStr=PParamDataTypeStr  OutMin=POutMin  OutMax=POutMax  OutDataTypeMode=Specify via dialog  OutDataType=POutDataTypeStr  OutDataTypeStr=POutDataTypeStr
  Sum : Sum  DisableCoverage=on  Inputs=++|  AccumDataTypeStr=SumAccumDataTypeStr  OutMin=SumOutMin  OutMax=SumOutMax  OutDataTypeMode=Specify via dialog  OutDataType=SumOutDataTypeStr  OutDataTypeStr=SumOutDataTypeStr
  y : Outport  OutDataType=OutDataTypeStr  InitialOutput=0
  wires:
  u/1 -> Sum/1, Integral Gain/1
  Proportional Gain/1 -> y/1
  Integral Gain/1 -> Integrator/1
  Integrator/1 -> Sum/2
  Sum/1 -> Proportional Gain/1

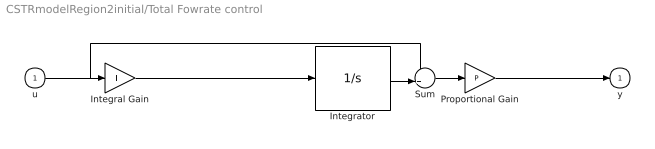
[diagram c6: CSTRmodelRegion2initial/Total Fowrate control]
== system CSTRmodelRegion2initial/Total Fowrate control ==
  u : Inport  OutDataType=OutDataTypeStr
  Integral Gain : Gain  DisableCoverage=on  Gain=I  ParamMin=IParamMin  ParamMax=IParamMax  ParameterDataTypeMode=Specify via dialog  ParameterDataType=IParamDataTypeStr  ParamDataTypeStr=IParamDataTypeStr  OutMin=IOutMin  OutMax=IOutMax  OutDataTypeMode=Specify via dialog  OutDataType=IOutDataTypeStr  OutDataTypeStr=IOutDataTypeStr
  Integrator : Integrator  DisableCoverage=on  InitialCondition=InitialConditionForIntegrator
  Proportional Gain : Gain  Gain=P  ParamMin=PParamMin  ParamMax=PParamMax  ParameterDataTypeMode=Specify via dialog  ParameterDataType=PParamDataTypeStr  ParamDataTypeStr=PParamDataTypeStr  OutMin=POutMin  OutMax=POutMax  OutDataTypeMode=Specify via dialog  OutDataType=POutDataTypeStr  OutDataTypeStr=POutDataTypeStr
  Sum : Sum  DisableCoverage=on  Inputs=++|  AccumDataTypeStr=SumAccumDataTypeStr  OutMin=SumOutMin  OutMax=SumOutMax  OutDataTypeMode=Specify via dialog  OutDataType=SumOutDataTypeStr  OutDataTypeStr=SumOutDataTypeStr
  y : Outport  OutDataType=OutDataTypeStr  InitialOutput=0
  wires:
  u/1 -> Sum/1, Integral Gain/1
  Proportional Gain/1 -> y/1
  Integral Gain/1 -> Integrator/1
  Integrator/1 -> Sum/2
  Sum/1 -> Proportional Gain/1

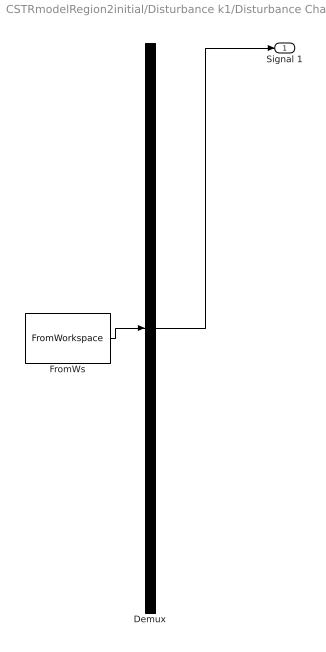
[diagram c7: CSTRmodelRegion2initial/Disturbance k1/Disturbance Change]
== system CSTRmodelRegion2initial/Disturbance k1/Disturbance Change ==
  Demux : Demux  Tag=STV Demux  Outputs=1
  FromWs : FromWorkspace  Tag=STV FromWs  VariableName=tuvar  SampleTime=0  SigBuilderData=DataTag0  VnvData=DataTag1
  Signal 1 : Outport  Tag=STV Outport  OutDataType=fixdt(1, 16)  OutScaling=2^0
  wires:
  FromWs/1 -> Demux/1
  Demux/1 -> Signal 1/1

== matlab function Self-optimizing 
Variable ==
function cs = fcn(Fa,Fb,V,cVector)


cain        =  2;
cbin        = 1.5;
Fmax        = 22;
k2          =  0.0140;
cb          =  cVector(2);

cs = (-cbin^2*Fa^2-Fa^2*cain*cbin+6*Fa*cain*k2*cb^2*V+2*Fa*cain*Fmax*cb-Fa*cain*Fmax*cbin+4*V*k2*cb^3*Fmax+4*V^2*k2^2*cb^4-2*cbin*Fmax^2*cb+Fmax^2*cb^2-4*V*k2*cb^2*cbin*Fmax+cbin^2*Fmax^2)/Fmax;
cs =cs/V;
